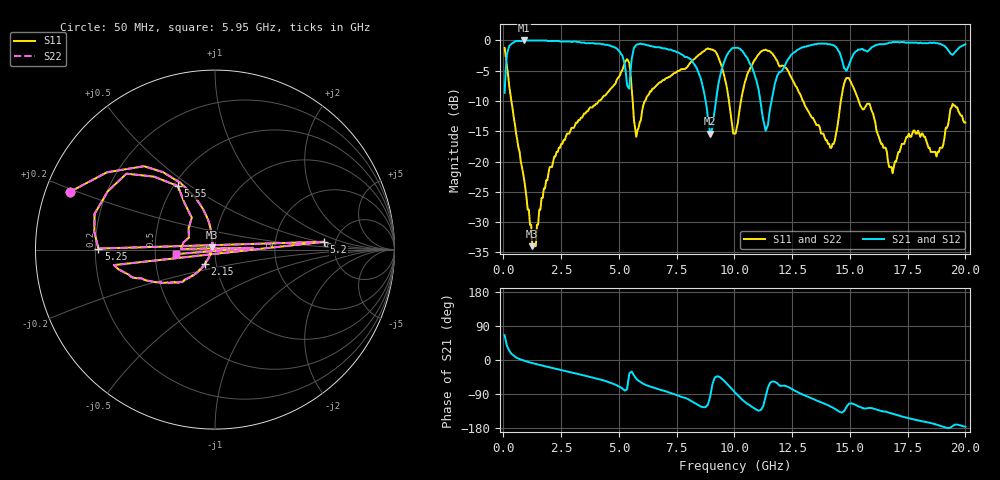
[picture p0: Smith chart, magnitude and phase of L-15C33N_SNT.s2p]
#	mhz	s	ma	r	50
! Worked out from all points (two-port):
!   400 points, 50 MHz to 20 GHz, reference 50 ohm
!   highest |S21| = 0.00 dB at 900 MHz (marker M1); lowest = -15.4 dB at 8.95 GHz (marker M2)
!   |S21| within 3 dB of the highest: 136 MHz to 5.185 GHz (5.049 GHz wide, 190 % of centre); 15.06 GHz to end of sweep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
!   lowest |S11| = -34.0 dB at 1.25 GHz (marker M3), VSWR 1.04, Z = 48.4 + j1.17 ohm
!   |S11| at or under -10 dB: 343.3 MHz to 4.131 GHz (3.788 GHz wide, 169 % of centre); 12.97 GHz to 14.61 GHz (1.64 GHz wide, 11.9 % of centre); 15.38 GHz to end of sweep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
!   |S22| runs from -34.0 to -1.2 dB; largest |S21 - S12| = 0
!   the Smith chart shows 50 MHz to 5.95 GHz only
!   S11 on the Smith chart (normalised r, x): 50 MHz: 0.07, +0.19; 2.15 GHz: 0.88, -0.15; 5.2 GHz: 4.05, +0.56; 5.25 GHz: 0.21, +0.00; 5.55 GHz: 0.53, +0.45; 5.95 GHz: 0.64, -0.03
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50  0.87 158.3  0.37 65.4  0.37 65.4  0.87 158.3
250  0.42 117.5  0.9 24.6  0.9 24.6  0.42 117.5
900  0.07 104.4  1 -2.0  1 -2.0  0.07 104.4
1250  0.02 143.0  1 -8.1  1 -8.1  0.02 143.0
2150  0.1 -125.0  0.99 -21.6  0.99 -21.6  0.1 -125.0
3400  0.23 -134.6  0.96 -39.6  0.96 -39.6  0.23 -134.6
5150  0.57 -171.3  0.75 -75.4  0.75 -75.4  0.57 -171.3
5200  0.61 4.1  0.69 -78.1  0.69 -78.1  0.61 4.1
5250  0.65 179.5  0.64 -80.7  0.64 -80.7  0.65 179.5
5550  0.41 120.3  0.7 -30.3  0.7 -30.3  0.41 120.3
5950  0.22 -173.4  0.94 -58.8  0.94 -58.8  0.22 -173.4
6700  0.44 -175.8  0.88 -76.8  0.88 -76.8  0.44 -175.8
6950  0.47 -179.6  0.86 -81.2  0.86 -81.2  0.47 -179.6
7000  0.48 -0.5  0.86 -82.2  0.86 -82.2  0.48 -0.5
7050  0.49 178.7  0.85 -83.2  0.85 -83.2  0.49 178.7
8950  0.85 105.1  0.17 -96.6  0.17 -96.6  0.85 105.1
10050  0.17 115.3  0.87 -87.0  0.87 -87.0  0.17 115.3
11350  0.84 90.9  0.18 -97.5  0.18 -97.5  0.84 90.9
13350  0.23 25.4  0.92 -101.6  0.92 -101.6  0.23 25.4
14950  0.49 8.8  0.62 -115.6  0.62 -115.6  0.49 8.8
16700  0.09 48.8  0.96 -139.1  0.96 -139.1  0.09 48.8
20000  0.21 -62.0  0.93 -176.1  0.93 -176.1  0.21 -62.0
